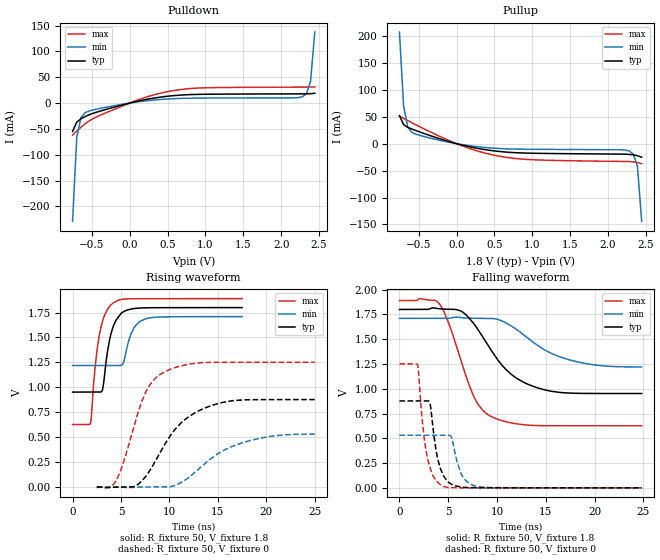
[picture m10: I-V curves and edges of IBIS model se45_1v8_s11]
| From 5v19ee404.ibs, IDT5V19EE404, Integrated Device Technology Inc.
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[Model]   se45_1v8_s11
Model_type   Output
Polarity   Non-Inverting
|   typ   min   max
C_comp   2pF   1.5pF   2.5pF
Vmeas = 0.9V
Rref = 50
Cref = 0
Vref = 0.9V
|   typ   min   max
[Voltage range]   1.8V   1.71V   1.89V
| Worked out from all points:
|   slope of the pulldown table from 0 to 0.27 V, typ, clamps not added: 32 ohm
|   slope of the pullup table from 0 to 0.27 V, typ, clamps not added: 31.6 ohm
|   rising waveform, R_fixture 50, V_fixture 1.8: 20-80 % time 981ps typ, 1.01ns min, 959ps max; typ from 0.952 V to 1.8 V
|   falling waveform, R_fixture 50, V_fixture 1.8: 20-80 % time 3.96ns typ, 4.76ns min, 2.69ns max; typ from 1.8 V to 0.952 V
|   rising waveform, R_fixture 50, V_fixture 0: 20-80 % time 3.91ns typ, 4.82ns min, 2.57ns max; typ from 0 V to 0.877 V
|   falling waveform, R_fixture 50, V_fixture 0: 20-80 % time 938ps typ, 983ps min, 929ps max; typ from 0.877 V to 0 V
[Pulldown]
|Voltage   I (typ)   I (min)   I (max)
|Note, modeling breaks down at 250mA and above.  This is well beyond the functional   |
|operating range of the device.  Should this scenario occur, catastrophic failure and   |
|possible damage to the device and/or board is of higher concern than the I-V curve   |
|behavior.  The IBIS checker will flag currents in excess of 10A with warnings.  Lines   |
|with currents in excess of 0.35 A have been commented out.  The points still remain|
|available to the user if the user desires to use them.   |
|-1.80000e+00   -2.52572e+01   -2.08112e+01   -3.26463e+01
|-1.74490e+00   -2.36799e+01   -1.95979e+01   -3.04476e+01
|-1.68980e+00   -2.21059e+01   -1.83872e+01   -2.82531e+01
|-1.63469e+00   -2.05356e+01   -1.71794e+01   -2.60635e+01
|-1.57959e+00   -1.89696e+01   -1.59750e+01   -2.38796e+01
|-1.52449e+00   -1.74087e+01   -1.47744e+01   -2.17024e+01
|-1.46939e+00   -1.58536e+01   -1.35783e+01   -1.95332e+01
|-1.41429e+00   -1.43055e+01   -1.23874e+01   -1.73739e+01
|-1.35918e+00   -1.27659e+01   -1.12027e+01   -1.52269e+01
|-1.30408e+00   -1.12368e+01   -1.00254e+01   -1.30956e+01
|-1.24898e+00   -9.72098e+00   -8.85722e+00   -1.09851e+01
|-1.19388e+00   -8.22246e+00   -7.70043e+00   -8.90351e+00
|-1.13878e+00   -6.74727e+00   -6.55830e+00   -6.86403e+00
|-1.08367e+00   -5.30512e+00   -5.43552e+00   -4.89135e+00
|-1.02857e+00   -3.91270e+00   -4.33946e+00   -3.03736e+00
|-9.73469e-01   -2.60169e+00   -3.28214e+00   -1.43100e+00
|-9.18367e-01   -1.43880e+00   -2.28475e+00   -3.94093e-01
|-8.63265e-01   -5.66865e-01   -1.38741e+00   -1.06939e-01
|-8.08163e-01   -1.52138e-01   -6.66903e-01   -7.19895e-02
-753.1mV  -54.82mA   -228.9mA   -62.01mA
-698mV    -36.89mA   -66.92mA   -54.09mA
-642.9mV  -30.52mA   -28.08mA   -46.79mA
-587.8mV  -26.13mA   -18.74mA   -40.17mA
-422.4mV  -17.04mA   -11.39mA   -25.78mA
73.47mV   2.606mA    1.636mA    4.206mA
569.4mV   14.28mA    8.482mA    23.96mA
1.01V     17.09mA    9.709mA    29.63mA
2.278V    17.85mA    12.06mA    30.89mA
2.333V    17.94mA    17.98mA    30.92mA
2.388V    18.19mA    42.4mA     30.98mA
2.443V    19.06mA    137.5mA    31.13mA
| 2.49796e+00   2.27208e-02   3.74787e-01   3.15041e-02
| 2.55306e+00   4.08756e-02   7.43068e-01   3.22551e-02
| 2.60816e+00   1.37566e-01   1.19023e+00   3.34916e-02
| 2.66327e+00   4.37819e-01   1.68221e+00   3.56718e-02
| 2.71837e+00   9.27501e-01   2.20139e+00   4.47213e-02
| 2.77347e+00   1.51885e+00   2.73835e+00   1.23384e-01
| 2.82857e+00   2.16314e+00   3.28769e+00   4.92594e-01
| 2.88367e+00   2.83803e+00   3.84607e+00   1.15125e+00
| 2.93878e+00   3.53242e+00   4.41129e+00   1.94102e+00
| 2.99388e+00   4.24015e+00   4.98190e+00   2.79125e+00
| 3.04898e+00   4.95754e+00   5.55682e+00   3.67438e+00
| 3.10408e+00   5.68219e+00   6.13525e+00   4.57781e+00
| 3.15918e+00   6.41253e+00   6.71663e+00   5.49491e+00
| 3.21429e+00   7.14740e+00   7.30048e+00   6.42176e+00
| 3.26939e+00   7.88598e+00   7.88646e+00   7.35591e+00
| 3.32449e+00   8.62763e+00   8.47428e+00   8.29574e+00
| 3.37959e+00   9.37188e+00   9.06370e+00   9.24008e+00
| 3.43469e+00   1.01184e+01   9.65453e+00   1.01881e+01
| 3.48980e+00   1.08667e+01   1.02466e+01   1.11392e+01
| 3.54490e+00   1.16168e+01   1.08398e+01   1.20928e+01
| 3.60000e+00   1.23684e+01   1.14340e+01   1.30487e+01
[Pullup]
|Voltage   I (typ)   I (min)   I (max)
|Note, modeling breaks down at 250mA and above.  This is well beyond the functional   |
|operating range of the device.  Should this scenario occur, catastrophic failure and   |
|possible damage to the device and/or board is of higher concern than the I-V curve   |
|behavior.  The IBIS checker will flag currents in excess of 10A with warnings.  Lines   |
|with currents in excess of 0.35 A have been commented out.  The points still remain|
|available to the user if the user desires to use them.   |
|-1.80000e+00   1.23492e+01   1.04530e+01   1.45809e+01
|-1.74490e+00   1.15979e+01   9.86061e+00   1.36224e+01
|-1.68980e+00   1.08480e+01   9.26940e+00   1.26656e+01
|-1.63469e+00   1.00998e+01   8.67956e+00   1.17108e+01
|-1.57959e+00   9.35349e+00   8.09124e+00   1.07584e+01
|-1.52449e+00   8.60944e+00   7.50468e+00   9.80872e+00
|-1.46939e+00   7.86800e+00   6.92013e+00   8.86233e+00
|-1.41429e+00   7.12967e+00   6.33794e+00   7.91994e+00
|-1.35918e+00   6.39506e+00   5.75851e+00   6.98248e+00
|-1.30408e+00   5.66501e+00   5.18238e+00   6.05131e+00
|-1.24898e+00   4.94068e+00   4.61027e+00   5.12833e+00
|-1.19388e+00   4.22372e+00   4.04313e+00   4.21650e+00
|-1.13878e+00   3.51650e+00   3.48228e+00   3.32063e+00
|-1.08367e+00   2.82280e+00   2.92962e+00   2.44927e+00
|-1.02857e+00   2.14888e+00   2.38803e+00   1.61954e+00
|-9.73469e-01   1.50615e+00   1.86206e+00   8.71510e-01
|-9.18367e-01   9.17564e-01   1.35944e+00   3.11233e-01
|-8.63265e-01   4.33414e-01   8.94316e-01   8.94593e-02
|-8.08163e-01   1.42396e-01   4.94089e-01   5.74619e-02
-753.1mV  52mA       207.1mA    51.2mA
-698mV    35.06mA    69.7mA     46.91mA
-642.9mV  30.25mA    30.46mA    42.81mA
-587.8mV  27.07mA    20.93mA    38.78mA
-312.2mV  13.24mA    9.215mA    19.54mA
73.47mV   -2.62mA    -1.732mA   -4.049mA
569.4mV   -14.56mA   -9.029mA   -23.39mA
1.065V    -17.95mA   -10.52mA   -30.19mA
2.278V    -19.91mA   -13.47mA   -33.25mA
2.333V    -20.75mA   -19.16mA   -33.68mA
2.388V    -22.37mA   -42.35mA   -34.85mA
2.443V    -25.08mA   -144mA     -37.25mA
| 2.49796e+00   -3.03122e-02   -4.72515e-01   -4.09753e-02
| 2.55306e+00   -4.85503e-02   -1.10341e+00   -4.57713e-02
| 2.60816e+00   -1.49867e-01   -1.94886e+00   -5.14012e-02
| 2.66327e+00   -5.72739e-01   -2.91646e+00   -5.79887e-02
| 2.71837e+00   -1.45030e+00   -3.95533e+00   -7.00790e-02
| 2.77347e+00   -2.61576e+00   -5.03908e+00   -1.50146e-01
| 2.82857e+00   -3.92793e+00   -6.15313e+00   -6.90731e-01
| 2.88367e+00   -5.32086e+00   -7.28879e+00   -1.99805e+00
| 2.93878e+00   -6.76320e+00   -8.44055e+00   -3.72340e+00
| 2.99388e+00   -8.23838e+00   -9.60470e+00   -5.63149e+00
| 3.04898e+00   -9.73678e+00   -1.07787e+01   -7.63318e+00
| 3.10408e+00   -1.12524e+01   -1.19607e+01   -9.69020e+00
| 3.15918e+00   -1.27812e+01   -1.31493e+01   -1.17833e+01
| 3.21429e+00   -1.43206e+01   -1.43434e+01   -1.39018e+01
| 3.26939e+00   -1.58683e+01   -1.55422e+01   -1.60388e+01
| 3.32449e+00   -1.74231e+01   -1.67451e+01   -1.81901e+01
| 3.37959e+00   -1.89838e+01   -1.79514e+01   -2.03526e+01
| 3.43469e+00   -2.05494e+01   -1.91609e+01   -2.25242e+01
| 3.48980e+00   -2.21193e+01   -2.03730e+01   -2.47033e+01
| 3.54490e+00   -2.36930e+01   -2.15876e+01   -2.68887e+01
| 3.60000e+00   -2.52699e+01   -2.28044e+01   -2.90795e+01
[Ramp]
|   typ   min   max
dV/dt_r   0.508/0.981n   0.294/1.014n   0.758/0.959n
dV/dt_f   0.518/4.015n   0.302/4.846n   0.769/2.729n
R_load =   50.0000
[Rising Waveform]
R_fixture = 50
V_fixture = 1.8   |Vcc_typ
V_fixture_min = 1.71 |Vcc_min
V_fixture_max = 1.89 |Vcc_max
C_fixture = 0.0p
| Time   typ   min   max
0s        951.9mV    1.218V     626.3mV
1.875ns   951.9mV    1.218V     648.3mV
2.27ns    951.9mV    1.218V     1.143V
2.793ns   951.8mV    1.218V     1.54V
3.084ns   972.5mV    1.218V     1.661V
4.292ns   1.633V     1.218V     1.853V
5.188ns   1.755V     1.235V     1.885V
6.25ns    1.789V     1.581V     1.889V
7.5ns     1.798V     1.686V     1.889V
17.5ns    1.8V       1.71V      1.89V
[Falling Waveform]
R_fixture = 50
V_fixture = 1.8   |Vcc_typ
V_fixture_min = 1.71 |Vcc_min
V_fixture_max = 1.89 |Vcc_max
C_fixture = 0.0p
| Time   typ   min   max
0s        1.8V       1.71V      1.89V
4.006ns   1.808V     1.71V      1.866V
5.013ns   1.802V     1.71V      1.672V
6.25ns    1.787V     1.718V     1.303V
7.63ns    1.655V     1.711V     919.8mV
9.412ns   1.387V     1.71V      719.6mV
11.55ns   1.138V     1.628V     653.7mV
14.31ns   1.004V     1.427V     627.9mV
18.76ns   953mV      1.26V      626.4mV
24.82ns   951.9mV    1.219V     626.3mV
[Rising Waveform]
R_fixture = 50
V_fixture = 0
C_fixture = 0.0p
| Time   typ   min   max
2.5ns     -112.9nV   55.92nV    -5.225mV
4.412ns   -2.046mV   8.164uV    50.67mV
5.185ns   -597.1uV   -2.334mV   226.6mV
6.363ns   4.382mV    -2.802mV   617.9mV
7.5ns     98.76mV    -512.6uV   940.3mV
9.178ns   369.1mV    -24.28uV   1.138V
11.32ns   652.7mV    50.69mV    1.217V
14.28ns   814.8mV    284.9mV    1.25V
18.8ns    876mV      476.9mV    1.251V
25ns      876.9mV    530.6mV    1.251V
[Falling Waveform]
R_fixture = 50
V_fixture = 0
C_fixture = 0.0p
| Time   typ   min   max
0s        876.9mV    531.2mV    1.251V
1.867ns   876.9mV    531.2mV    1.239V
2.513ns   876.9mV    531.2mV    520mV
3.07ns    868.1mV    531.2mV    228.6mV
3.816ns   345.3mV    531.2mV    68.11mV
4.514ns   124.2mV    531.2mV    14.14mV
5.288ns   38.63mV    518.3mV    1.607mV
6.314ns   8.056mV    144.8mV    494.5uV
7.717ns   1.062mV    20.07mV    327.3uV
24.82ns   27.16uV    52.99uV    14.98uV
